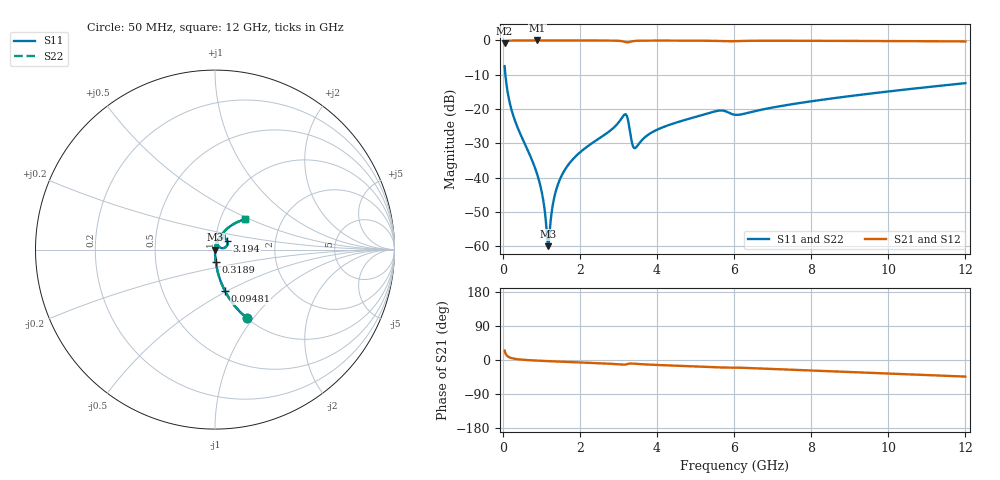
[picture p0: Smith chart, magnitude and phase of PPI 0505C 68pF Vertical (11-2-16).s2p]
# GHz S MA R 50
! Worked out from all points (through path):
!   1601 points, 50 MHz to 12 GHz, reference 50 ohm
!   highest |S21| = -0.01 dB at 901.4 MHz (marker M1); lowest = -0.9 dB at 50 MHz (marker M2)
!   group delay of S21, straight-line fit = 10.5 ps
!   lowest |S11| = -59.9 dB at 1.178 GHz (marker M3), VSWR 1.00, Z = 50.1 - j0.0137 ohm
!   |S11| at or under -10 dB: 69.84 MHz to end of sweep
!   |S22| runs from -59.9 to -7.5 dB; largest |S21 - S12| = 0
!   S11 on the Smith chart (normalised r, x): 50 MHz: 1.00, -0.93; 94.81 MHz: 1.00, -0.49; 318.9 MHz: 1.00, -0.14; 3.194 GHz: 1.14, +0.11; 12 GHz: 1.31, +0.47
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0.05  0.4223 -65.1  0.9062 24.9  0.9062 24.9  0.4223 -65.1
0.0948125  0.2376 -76.4  0.971 13.5  0.971 13.5  0.2376 -76.4
0.1844375  0.1225 -83.2  0.992 6.6  0.992 6.6  0.1225 -83.2
0.318875  0.06775 -86.4  0.9971 3.1  0.9971 3.1  0.06775 -86.4
0.9014375  0.01092 -87.0  0.999 -1.7  0.999 -1.7  0.01092 -87.0
1.028406  0.005612 -82.6  0.999 -2.3  0.999 -2.3  0.005612 -82.6
1.140437  0.001697 -57.2  0.9989 -2.8  0.9989 -2.8  0.001697 -57.2
1.177781  0.001008 -7.8  0.9989 -3.0  0.9989 -3.0  0.001008 -7.8
1.215125  0.001555 45.8  0.9989 -3.2  0.9989 -3.2  0.001555 45.8
1.334625  0.005099 74.2  0.9988 -3.7  0.9988 -3.7  0.005099 74.2
1.469062  0.009048 78.6  0.9987 -4.3  0.9987 -4.3  0.009048 78.6
1.700594  0.01543 80.2  0.9985 -5.2  0.9985 -5.2  0.01543 80.2
2.044156  0.02447 80.0  0.9981 -6.6  0.9981 -6.6  0.02447 80.0
3.194344  0.08363 36.9  0.9426 -11.8  0.9426 -11.8  0.08363 36.9
3.366125  0.03039 21.9  0.9737 -9.5  0.9737 -9.5  0.03039 21.9
3.425875  0.02697 41.6  0.9828 -10.0  0.9828 -10.0  0.02697 41.6
4.038312  0.05109 72.7  0.9948 -13.2  0.9948 -13.2  0.05109 72.7
5.561937  0.0941 62.1  0.9815 -19.5  0.9815 -19.5  0.0941 62.1
6.025  0.0826 56.3  0.9767 -19.9  0.9767 -19.9  0.0826 56.3
8.019156  0.1303 60.6  0.9872 -27.7  0.9872 -27.7  0.1303 60.6
10.01331  0.1809 53.3  0.9792 -35.6  0.9792 -35.6  0.1809 53.3
12  0.2387 45.3  0.9664 -43.8  0.9664 -43.8  0.2387 45.3
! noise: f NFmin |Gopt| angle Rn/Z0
0.05  0.000379  0.8612  0.4272  0.000585
1.372  0.003903  0.6682  3.483  0.002257
2.701  0.008959  0.7088  6.75  0.006031
4.031  0.0122  0.6857  10.07  0.00748
5.36  0.02047  0.743  13.4  0.01577
6.682  0.02038  0.6889  16.54  0.01248
8.012  0.01773  0.5963  19.2  0.00786
9.341  0.01889  0.5679  21.94  0.007626
10.67  0.02069  0.5553  24.66  0.007982
12  0.02279  0.55  27.33  0.008574
